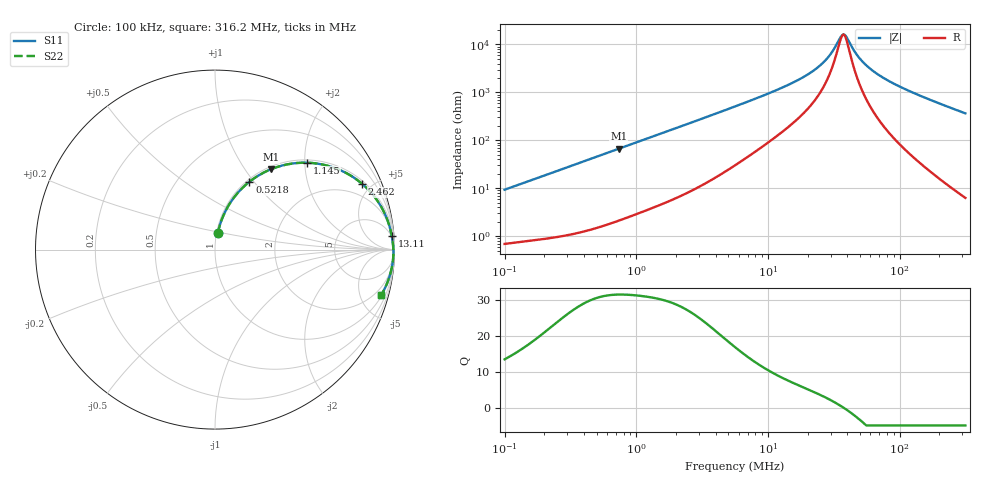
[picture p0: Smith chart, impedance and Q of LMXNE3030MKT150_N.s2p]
! LMXNE3030MKT150_N  S-PARAMETER MODEL  ( General Type )
! Model Generated by TAIYO YUDEN Corporation (http://www.ty-top.com)
! Version 1.0
! TAIYO YUDEN Control No. 191023NI43SB-FBB
! Copyright(c) 2019 TAIYO YUDEN CO.,LTD. All Rights Reserved.
! Product Description (link to TY-COMPAS)
! https://ds.yuden.co.jp/TYCOMPAS/or/detail?pn=LMXNE3030MKT150MN&u=M
! Products Name : Inductors
! Characteristics :
!  Inductance : 15 uH , SRF(min) : 26 MHz , DC Resistance(max) : 0.54 Ohm
!  Rated Current : Saturation :530 mA , Temp Rise : 570 mA
!  Case Size : 3.0 x 3.0 / 0.118 x 0.118 [mm/inch] , Thickness : 1.2 / 0.047 [mm/inch]
!  (Conditions: Temperature = 25 degC , DC Bias Current/Voltage = 0A / 0V)
! External Node Assignments :
!  1  o---GGG---o  2
! GND o---------o GND
! Frequency Range : 0.1MHz  -  316.199832MHz  [ 402 STEP ]
# MHz S RI R 50
! Freq[MHz].  S11 Real  S11 Imag  S21 Real  S21 Imag  S12 Real  S12 Imag  S22 Real  S22 Imag
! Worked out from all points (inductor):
!   401 points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, 100 kHz to 316.2 MHz, reference 50 ohm
!   read as one part in series: L = 14.7 uH near 104.1 kHz
!   highest Q = 31.6 at 734.9 kHz (marker M1), where L = 14.4 uH
!   self-resonance near 37.37 MHz
!   S11 on the Smith chart (normalised r, x): 100 kHz: 1.01, +0.19; 521.8 kHz: 1.03, +0.95; 1.145 MHz: 1.07, +2.06; 2.462 MHz: 1.16, +4.40; 13.11 MHz: 4, +26; 316.2 MHz: 1.13, -7.29
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0.1  0.0152 0.091  0.9848 -0.091  0.9848 -0.091  0.0152 0.091
0.219405  0.0469 0.1901  0.9531 -0.1901  0.9531 -0.1901  0.0469 0.1901
0.385695  0.1185 0.3063  0.8815 -0.3063  0.8815 -0.3063  0.1185 0.3063
0.521786  0.1916 0.3777  0.8084 -0.3777  0.8084 -0.3777  0.1916 0.3777
0.734921  0.3126 0.448  0.6874 -0.448  0.6874 -0.448  0.3126 0.448
1.144823  0.5149 0.484  0.4851 -0.484  0.4851 -0.484  0.5149 0.484
1.487603  0.6365 0.4648  0.3635 -0.4648  0.3635 -0.4648  0.6365 0.4648
2.461698  0.8204 0.3659  0.1796 -0.3659  0.1796 -0.3659  0.8204 0.3659
5.623165  0.9526 0.1849  0.0474 -0.1849  0.0474 -0.1849  0.9526 0.1849
13.1062  0.9849 0.0751  0.0151 -0.0751  0.0151 -0.0751  0.9849 0.0751
21.68824  0.9909 0.0353  0.00907 -0.0353  0.00907 -0.0353  0.9909 0.0353
28.18209  0.9927 0.018  0.00729 -0.018  0.00729 -0.018  0.9927 0.018
31.16898  0.9932 0.0116  0.00679 -0.0116  0.00679 -0.0116  0.9932 0.0116
35.88988  0.9937 0.00265  0.00626 -0.00265  0.00626 -0.00265  0.9937 0.00265
37.36559  0.9939 9.52e-05  0.00615 -9.52e-05  0.00615 -9.52e-05  0.9939 9.52e-05
39.69369  0.994 -0.00375  0.00601 0.00375  0.00601 0.00375  0.994 -0.00375
46.63594  0.9942 -0.0142  0.00583 0.0142  0.00583 0.0142  0.9942 -0.0142
53.69948  0.9941 -0.0237  0.00593 0.0237  0.00593 0.0237  0.9941 -0.0237
65.68544  0.9935 -0.0382  0.00653 0.0382  0.00653 0.0382  0.9935 -0.0382
83.65039  0.9918 -0.0577  0.00817 0.0577  0.00817 0.0577  0.9918 -0.0577
147.0501  0.9813 -0.1179  0.0187 0.1179  0.0187 0.1179  0.9813 -0.1179
316.1998  0.9264 -0.2527  0.0736 0.2527  0.0736 0.2527  0.9264 -0.2527
